FUNCTION_BLOCK Example28b_zoneloading //2x1 flyways 2 xbots (actual physical) - ZoneCtrl, FenceCtrl, GetStatus
VAR_INPUT
	Execute : BOOL;
	UserFinishedAddingXbot : BOOL;
END_VAR
VAR_OUTPUT
	UserCanAddXbot : BOOL;
	Done : BOOL;
END_VAR
VAR_IN_OUT
	PM_Controller : PMControllerType;	// the planar motor controller to use
END_VAR
VAR
	PMC_XYMotion1 : PMC_XYMotion;
	PMC_Zone_ZoneCtrl1 : PMC_Zone_ZoneCtrl;
	PMC_Zone_ZoneCtrl2 : PMC_Zone_ZoneCtrl;
	PMC_Zone_Fencing1 : PMC_Zone_Fencing; 
	PMC_Zone_GetStatus1 : PMC_Zone_GetStatus;
	PMC_XYMotion2 : PMC_XYMotion;
END_VAR

//2x1 flyways 2 xbots (actual physical) - ZoneCtrl, FenceCtrl, GetStatus

IF NOT(Execute) THEN
	UserFinishedAddingXbot := FALSE;
END_IF; 

//move xbot 1 to side
PMC_XYMotion1(Execute := Execute,cmdLB := 1,XbotID := 1,Mode := 0,Type_ := 0,PosX := 0.06,PosY := 0.18,EndVel := 0,MaxVel := 1,MaxAcc := 10,PM_Controller := PM_Controller);

//deactivate zone 2 (flyway 2)
PMC_Zone_ZoneCtrl1(Execute := PMC_XYMotion1.Done,ZoneID := 2,Level := 0,PM_Controller := PM_Controller);

//tell user that they can now put the xbot into the zone
UserCanAddXbot := PMC_Zone_ZoneCtrl1.Done;

//activate zone once user says they are done adding the xbot
PMC_Zone_ZoneCtrl2(Execute := UserFinishedAddingXbot AND PMC_Zone_ZoneCtrl1.Done,ZoneID := 2,Level := 1,PM_Controller := PM_Controller);

//read zone info
PMC_Zone_GetStatus1(Execute := PMC_Zone_ZoneCtrl2.Done,ZoneID := 2,PM_Controller := PM_Controller);

//turn off fence on zone 2
PMC_Zone_Fencing1(Execute := PMC_Zone_GetStatus1.Done,ZoneID := 2,Level := 0,PM_Controller := PM_Controller);

//move xbot in zone 2 to side
PMC_XYMotion2(Execute := PMC_Zone_Fencing1.Done,cmdLB := 8,XbotID := PMC_Zone_GetStatus1.XbotIDs[0],Mode := 0,Type_ := 2,PosX := 0.06,PosY := 0.06,EndVel := 0,MaxVel := 1,MaxAcc := 10,PM_Controller := PM_Controller);

Done := PMC_XYMotion2.Done;

END_FUNCTION_BLOCK
